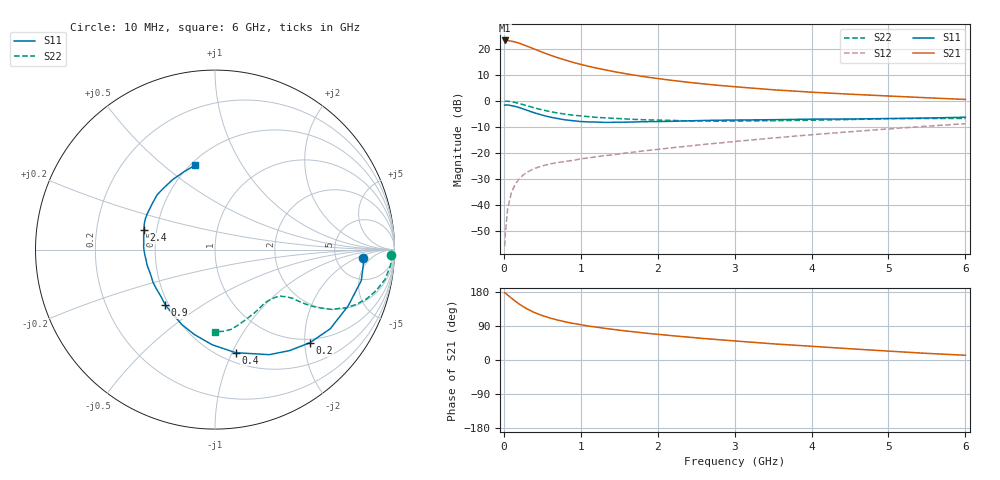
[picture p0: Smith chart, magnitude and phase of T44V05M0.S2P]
! Infineon Technologies  Discrete & RF Semiconductors
! BFR182T
! Si NPN RF Bipolar Junction Transistor in SC75
! VCE = 4 V  IC = 5 mA
! Common Emitter S-Parameters:  October  1999
# GHz  S  MA  R  50
!  f  S11  S21  S12  S22
! GHz  MAG  ANG  MAG  ANG  MAG  ANG  MAG  ANG
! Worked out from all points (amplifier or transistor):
!   36 points, 10 MHz to 6 GHz, reference 50 ohm
!   highest |S21| = 23.2 dB at 10 MHz (marker M1)
!   |S21| within 3 dB of that: start of sweep to 370.4 MHz
!   unconditionally stable (mu >= 1): 1.406 GHz to 4.028 GHz
!   at 250 MHz: K = 0.28, MSG = 25.1 dB, |S12| = -28.6 dB
!   at 1.4 GHz: K = 1.00, MSG = 16.1 dB, |S12| = -20.8 dB
!   at 6 GHz: K = 0.84, MSG = 4.7 dB, |S12| = -8.8 dB
!   lowest NFmin = 1.20 dB at 450 MHz
!   S11 on the Smith chart (normalised r, x): 10 MHz: 10, -3; 200 MHz: 0.92, -2.11; 400 MHz: 0.59, -1.03; 900 MHz: 0.48, -0.36; 2.4 GHz: 0.42, +0.11; 6 GHz: 0.53, +0.65
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0.01  0.8257 -3.4  14.49 177.4  0.0016 75.5  0.9825 -1.7
0.02  0.8323 -3.2  14.45 176.7  0.0029 95.5  0.9814 -2.0
0.05  0.8334 -11.9  14.45 171.2  0.0085 85.4  0.9826 -5.1
0.1  0.8056 -22.9  14.03 163.1  0.0175 80.2  0.9615 -10.0
0.15  0.779 -34.5  13.49 154.9  0.025 72.4  0.9262 -14.3
0.2  0.7407 -44.5  12.83 147.6  0.0316 70.1  0.8883 -18.0
0.25  0.6993 -53.6  12.03 141.1  0.0371 64.6  0.8453 -21.1
0.3  0.6587 -62.7  11.28 135.1  0.0424 61.9  0.8056 -23.6
0.4  0.5856 -78.7  9.854 125.0  0.0502 57.1  0.7284 -27.2
0.5  0.5301 -91.8  8.605 117.3  0.0561 54.4  0.6698 -29.0
0.6  0.4867 -103.7  7.576 110.7  0.0609 53.5  0.6208 -30.4
0.7  0.4562 -114.0  6.751 105.4  0.065 52.0  0.5829 -31.1
0.9  0.414 -132.0  5.491 96.7  0.0717 52.6  0.5288 -31.9
1.1  0.3929 -146.3  4.622 89.6  0.0797 53.5  0.4962 -32.7
1.3  0.3849 -158.2  3.989 83.9  0.088 54.7  0.4713 -33.7
1.6  0.3885 -172.0  3.289 76.3  0.0996 56.6  0.4464 -35.4
2.2  0.4042 169.4  2.459 63.9  0.1257 59.8  0.4191 -41.2
2.4  0.4115 164.7  2.269 60.3  0.1348 60.6  0.412 -43.5
3.5  0.4333 143.9  1.631 42.7  0.1925 61.3  0.4147 -57.3
4.5  0.4469 129.1  1.341 29.7  0.254 58.9  0.4368 -71.5
5.5  0.4669 111.6  1.144 17.5  0.3252 54.5  0.4578 -84.4
6  0.4834 103.1  1.062 12.5  0.3632 51.2  0.4568 -89.8
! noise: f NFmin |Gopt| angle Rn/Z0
0.45  1.2  0.27  37  0.3
0.9  1.3  0.25  75  0.23
1.8  1.9  0.21  145  0.2
